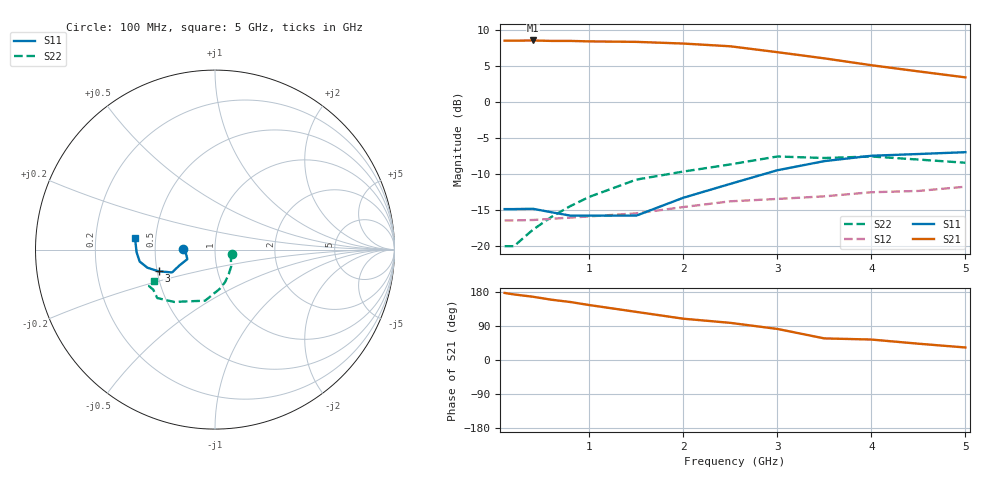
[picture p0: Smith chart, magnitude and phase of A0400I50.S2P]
!  MSA-0400 S AND NOISE PARAMETERS
!  Id=50mA  LAST UPDATED 07-22-92
# ghz s ma r 50
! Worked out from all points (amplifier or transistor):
!   14 points, 100 MHz to 5 GHz, reference 50 ohm
!   highest |S21| = 8.6 dB at 400 MHz (marker M1)
!   |S21| within 3 dB of that: start of sweep to 3.768 GHz
!   unconditionally stable (mu >= 1): start of sweep to 2.371 GHz
!   at 400 MHz: K = 1.35, MAG = 9.0 dB, |S12| = -16.4 dB
!   at 2 GHz: K = 1.07, MAG = 9.7 dB, |S12| = -14.6 dB
!   at 5 GHz: K = 0.93, MSG = 7.6 dB, |S12| = -11.7 dB
!   lowest NFmin = 6.10 dB at 100 MHz
!   S11 on the Smith chart (normalised r, x): 100 MHz: 0.69, +0.00; 3 GHz: 0.51, -0.14; 5 GHz: 0.38, +0.06
0.1  0.181 179.0  2.68 177.0  0.151 1.0  0.1 -13.0
0.2  0.181 180.0  2.68 173.0  0.151 3.0  0.1 -28.0
0.4  0.182 180.0  2.69 167.0  0.152 5.0  0.13 -46.0
0.6  0.172 -177.0  2.67 159.0  0.155 8.0  0.16 -62.0
0.8  0.163 -173.0  2.67 153.0  0.158 9.0  0.19 -73.0
1  0.163 -171.0  2.65 145.0  0.161 10.0  0.22 -83.0
1.5  0.163 -161.0  2.63 127.0  0.169 16.0  0.29 -101.0
2  0.217 -156.0  2.56 109.0  0.187 18.0  0.33 -119.0
2.5  0.271 -152.0  2.45 98.0  0.205 24.0  0.37 -128.0
3  0.337 -159.0  2.23 82.0  0.213 24.0  0.42 -140.0
3.5  0.39 -165.0  2.02 57.0  0.222 23.0  0.41 -147.0
4  0.425 -171.0  1.81 54.0  0.237 21.0  0.42 -151.0
4.5  0.437 -178.0  1.64 43.0  0.242 19.0  0.4 -152.0
5  0.45 172.0  1.49 33.0  0.259 17.0  0.38 -153.0
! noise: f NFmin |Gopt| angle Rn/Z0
0.1  6.1  0.13  180  0.63
0.5  6.2  0.14  -180  0.63
1  6.4  0.15  -178  0.63
2  7.1  0.2  -170  0.61
